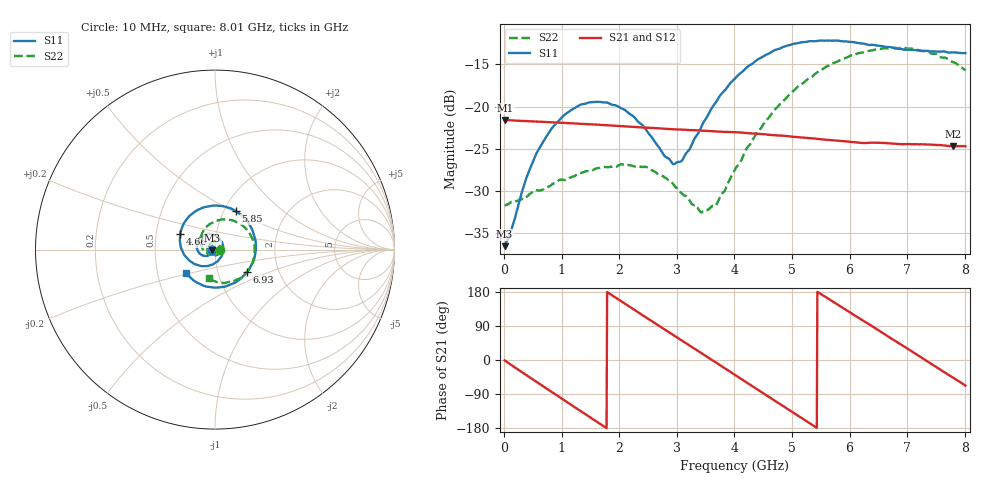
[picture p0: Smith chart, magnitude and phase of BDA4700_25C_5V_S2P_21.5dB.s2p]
!Agilent Technologies,E5071B,MY42404982,A.09.10
!Date: Mon Oct 20 13:37:11 2025
!Data & Calibration Information:
!Freq	S11:SOLT2(ON)	S21:SOLT2(ON)	S12:SOLT2(ON)	S22:SOLT2(ON)
# Hz S RI R 50
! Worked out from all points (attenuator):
!   801 points, 10 MHz to 8.01 GHz, reference 50 ohm
!   highest |S21| = -21.59 dB at 20 MHz (marker M1); lowest = -24.7 dB at 7.8 GHz (marker M2)
!   lowest |S11| = -36.5 dB at 10 MHz (marker M3), VSWR 1.03, Z = 48.5 - j0.13 ohm
!   |S11| at or under -10 dB: start of sweep to end of sweep
!   |S22| runs from -32.5 to -13.0 dB; largest |S21 - S12| = 0.00065
!   S11 on the Smith chart (normalised r, x): 10 MHz: 0.97, -0.00; 4.66 GHz: 0.67, +0.12; 5.85 GHz: 1.13, +0.52; 6.93 GHz: 1.38, -0.36; 8.01 GHz: 0.70, -0.19
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1e7  -0.0149 -0.00134  0.0833 -0.00179  0.0833 -0.00189  0.0261 -0.000838
2e7  -0.0152 -0.00209  0.0832 -0.00315  0.0833 -0.00346  0.026 -0.00109
3.8e8  -0.0261 -0.0263  0.0636 -0.0517  0.0636 -0.0518  0.0213 -0.0197
5.9e8  -0.0423 -0.0353  0.0403 -0.0707  0.0403 -0.0707  0.0134 -0.029
1e9  -0.0827 -0.024  -0.0161 -0.0785  -0.0162 -0.0785  -0.0148 -0.0339
1.35e9  -0.1022 0.0128  -0.0575 -0.0541  -0.0576 -0.0542  -0.0364 -0.0177
2.07e9  -0.0435 0.0862  -0.0672 0.0366  -0.0672 0.0366  -0.0301 0.0339
2.68e9  0.0375 0.0441  -0.00165 0.0743  -0.00167 0.0743  0.0138 0.0372
2.93e9  0.0458 0.00235  0.0291 0.0674  0.0291 0.0673  0.0254 0.024
3.06e9  0.0424 -0.0208  0.043 0.0591  0.0427 0.0592  0.0279 0.0139
3.44e9  -0.00416 -0.0776  0.069 0.0208  0.0691 0.0207  0.0184 -0.015
3.69e9  -0.0554 -0.092  0.0705 -0.00959  0.0706 -0.00982  -7.47e-05 -0.0264
4.01e9  -0.1276 -0.0718  0.0546 -0.0446  0.0546 -0.0445  -0.0331 -0.0262
4.66e9  -0.1941 0.0848  -0.0158 -0.0658  -0.0156 -0.0659  -0.0804 0.0456
5.35e9  -0.0533 0.2376  -0.064 -0.00999  -0.0641 -0.0102  -0.0153 0.1491
5.85e9  0.1144 0.215  -0.0482 0.0398  -0.0482 0.0398  0.0977 0.1625
6.25e9  0.2082 0.1099  -0.0134 0.0593  -0.0128 0.0595  0.1817 0.1051
6.68e9  0.2203 -0.0447  0.0294 0.0529  0.0295 0.0529  0.2205 -0.00238
6.93e9  0.1785 -0.1246  0.0477 0.0361  0.0478 0.036  0.2117 -0.0711
7.36e9  0.0469 -0.2077  0.0594 -0.00462  0.0594 -0.00472  0.1369 -0.1621
7.8e9  -0.1075 -0.1796  0.0396 -0.0425  0.0396 -0.0427  0.0178 -0.182
8.01e9  -0.1611 -0.1302  0.0223 -0.0538  0.0224 -0.0538  -0.0326 -0.1607
